FUNCTION_BLOCK Example24b_autoloading_receiving //1 flyway 1 xbot (actual physical) - autoloading delete,create,activate,holdforzoneready,loadingzoneclear 
VAR_INPUT
	Execute : BOOL;
END_VAR
VAR_OUTPUT
	Done : BOOL;
END_VAR
VAR_IN_OUT
	PM_Controller : PMControllerType;	// the planar motor controller to use
END_VAR
VAR
	PMC_AutoLoadingZone_Delete1 : PMC_AutoLoadingZone_Delete;
	PMC_AutoLoadingZone_Create1 : PMC_AutoLoadingZone_Create;
	PMC_AutoLoadingZone_Activate1 : PMC_AutoLoadingZone_Activate;
	PMC_AutoLoadingZone_HoldForZoneReady1 : PMC_AutoLoadingZone_HoldForZoneReady;
	PMC_XYMotion1 : PMC_XYMotion;
	PMC_AutoLoadingZone_LoadingZoneClear1 : PMC_AutoLoadingZone_LoadingZoneClear;
END_VAR

//1 flyway 1 xbot (actual physical) - autoloading delete,create,activate,holdforzoneready,loadingzoneclear

//delete any existing zones
PMC_AutoLoadingZone_Delete1(Execute := Execute,ZoneID := 0,PM_Controller := PM_Controller);

//create an autoloading loading zone on the top left edge (75,240) of the flyway
PMC_AutoLoadingZone_Create1(Execute := PMC_AutoLoadingZone_Delete1.Done,ZoneID := 1,ZoneMode := 1,UnloadingMode := 0,
					ZoneCenterX := 0.075,ZoneCenterY := 0.24,ZoneLength := 0.12,ZoneWidth := 0.15,MaxXbotSizeX := 0.12,MaxXbotSizeY := 0.12,
					MaxVel := 2,MaxAcc := 10,MaxHeight := 0,PM_Controller := PM_Controller);

//activate the loading zone
PMC_AutoLoadingZone_Activate1(Execute := PMC_AutoLoadingZone_Create1.Done,ZoneID := 1,PM_Controller := PM_Controller);

//hold until the zone is ready (xbot is in the zone and is ready to move out of the zone
PMC_AutoLoadingZone_HoldForZoneReady1(Execute := PMC_AutoLoadingZone_Activate1.Done,ZoneID := 1,PM_Controller := PM_Controller);

//move xbot out of the zone
PMC_XYMotion1(Execute := PMC_AutoLoadingZone_HoldForZoneReady1.Done,cmdLB := 1,XbotID := PMC_AutoLoadingZone_HoldForZoneReady1.xbotID,Mode := 0,Type_ := 1,PosX := 0.18,PosY := 0.06,EndVel := 0,MaxVel := 1,MaxAcc := 10,PM_Controller := PM_Controller);

//tell the loading zone that the xbot has moved clear 
PMC_AutoLoadingZone_LoadingZoneClear1(Execute := PMC_XYMotion1.Done,ZoneID := 1,PM_Controller := PM_Controller);

Done := PMC_AutoLoadingZone_LoadingZoneClear1.Done;

END_FUNCTION_BLOCK
